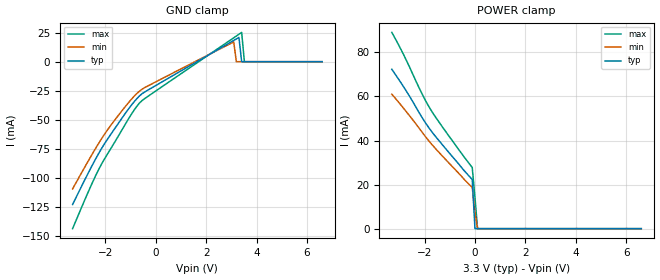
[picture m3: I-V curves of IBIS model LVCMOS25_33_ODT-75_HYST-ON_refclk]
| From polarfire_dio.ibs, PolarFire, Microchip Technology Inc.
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|   Model LVCMOS25_33_ODT-75_HYST-ON_refclk
[Model]   LVCMOS25_33_ODT-75_HYST-ON_refclk
Model_type   Input
Vinl =   0.7
Vinh =   1.7
|   typ   min   max
C_comp   5.210e-12   5.210e-12   5.520e-12
[Temperature Range]  25C   100C   -40C
[Voltage Range]  3.3   3.135   3.465
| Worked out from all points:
|   POWER clamp passes 1 mA (typ) near -0.00 V on its own axis
[GND Clamp]
| Voltage   I(typ)   I(min)   I(max)
-3.3V     -123.2mA   -109.7mA   -144.1mA
-2.599V   -92.62mA   -82.57mA   -108.4mA
-2.166V   -75.4mA    -66.93mA   -88.86mA
-1.191V   -44.06mA   -38.24mA   -53.25mA
-758mV    -32.03mA   -27.6mA    -38.64mA
-541.4mV  -27.59mA   -23.7mA    -33.48mA
3.094V    18.35mA    17.07mA    20.62mA
3.197V    19.64mA    0A         22.15mA
3.3V      20.93mA    0A         23.68mA
3.408V    0A         0A         25.28mA
3.517V    0A         0A         0A
6.6V      0A         0A         0A
[POWER Clamp]
| Voltage   I(typ)   I(min)   I(max)
-3.3V     72.33mA    61mA       89.06mA
-2.815V   64.08mA    54.38mA    78.57mA
-2.166V   51.69mA    44.81mA    62.68mA
-1.841V   45.97mA    39.97mA    55.62mA
-1.299V   38.16mA    33.02mA    46.29mA
-108.3mV  22.29mA    18.72mA    27.73mA
0V        0A         7.284mA    14.09mA
103.1mV   0A         0A         0A
6.6V      0A         0A         0A
